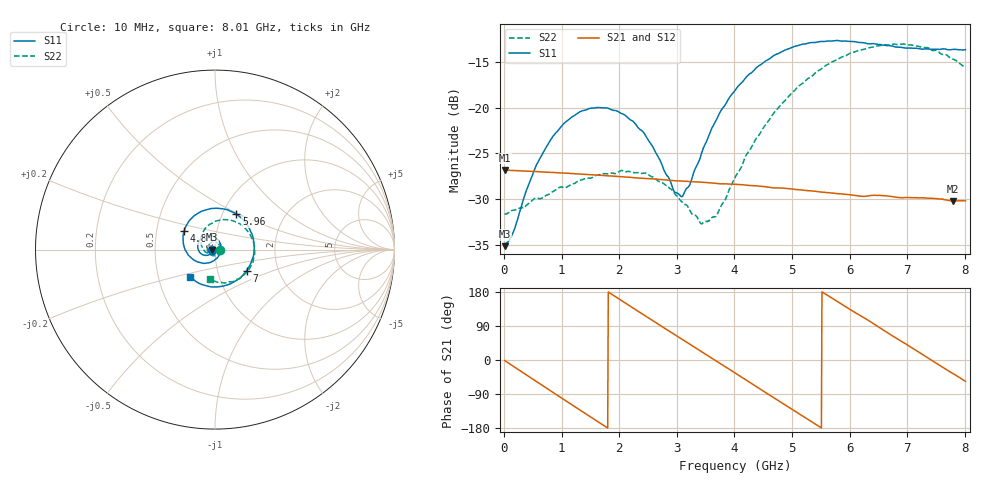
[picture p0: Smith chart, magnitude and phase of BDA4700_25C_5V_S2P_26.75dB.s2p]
!Agilent Technologies,E5071B,MY42404982,A.09.10
!Date: Mon Oct 20 13:39:58 2025
!Data & Calibration Information:
!Freq	S11:SOLT2(ON)	S21:SOLT2(ON)	S12:SOLT2(ON)	S22:SOLT2(ON)
# Hz S RI R 50
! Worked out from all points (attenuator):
!   801 points, 10 MHz to 8.01 GHz, reference 50 ohm
!   highest |S21| = -26.82 dB at 10 MHz (marker M1); lowest = -30.2 dB at 7.8 GHz (marker M2)
!   lowest |S11| = -35.2 dB at 10 MHz (marker M3), VSWR 1.04, Z = 48.3 - j0.102 ohm
!   |S11| at or under -10 dB: start of sweep to end of sweep
!   |S22| runs from -32.7 to -13.0 dB; largest |S21 - S12| = 0.00038
!   S11 on the Smith chart (normalised r, x): 10 MHz: 0.97, -0.00; 4.8 GHz: 0.69, +0.15; 5.96 GHz: 1.16, +0.48; 7 GHz: 1.38, -0.34; 8.01 GHz: 0.73, -0.23
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1e7  -0.0174 -0.00105  0.0456 -0.000973  0.0456 -0.00104  0.0261 -0.000789
1.5e8  -0.0184 -0.00909  0.0436 -0.0121  0.0436 -0.0121  0.0264 -0.00716
4.3e8  -0.0284 -0.0253  0.0324 -0.031  0.0325 -0.0309  0.0196 -0.0226
7.1e8  -0.0491 -0.0326  0.0141 -0.0421  0.014 -0.0421  0.00522 -0.0324
1.35e9  -0.0956 0.0061  -0.0306 -0.0305  -0.0306 -0.0305  -0.036 -0.0178
2.08e9  -0.051 0.0761  -0.0372 0.019  -0.0372 0.019  -0.0297 0.0335
2.42e9  -0.00594 0.073  -0.0203 0.0357  -0.0203 0.0357  -0.00495 0.0434
2.68e9  0.0215 0.049  -0.0031 0.0404  -0.0031 0.0404  0.0128 0.0374
2.95e9  0.0331 0.0112  0.0148 0.037  0.0148 0.0369  0.0251 0.0233
3.1e9  0.0304 -0.0119  0.0234 0.0319  0.0234 0.032  0.028 0.0115
3.41e9  0.00297 -0.0534  0.0358 0.0158  0.0358 0.0158  0.0203 -0.0115
3.54e9  -0.0157 -0.0662  0.0381 0.00757  0.0381 0.00752  0.0129 -0.0202
3.7e9  -0.045 -0.0748  0.0383 -0.00278  0.0383 -0.0029  -0.000747 -0.0259
4.01e9  -0.1061 -0.0642  0.0315 -0.0213  0.0315 -0.0213  -0.0323 -0.0257
4.8e9  -0.1722 0.1018  -0.0128 -0.034  -0.0127 -0.034  -0.078 0.0672
5.35e9  -0.0688 0.2157  -0.0336 -0.00972  -0.0336 -0.0098  -0.0152 0.1479
5.96e9  0.1191 0.1971  -0.0248 0.0224  -0.0249 0.0223  0.1217 0.1512
6.68e9  0.2175 -0.0148  0.0113 0.0307  0.0113 0.0307  0.2197 -0.000102
7e9  0.1758 -0.1172  0.0246 0.0207  0.0247 0.0206  0.2029 -0.0857
7.41e9  0.0597 -0.1994  0.0319 0.000359  0.0319 0.000285  0.1259 -0.1647
7.8e9  -0.0769 -0.1933  0.0248 -0.0182  0.0248 -0.0184  0.0202 -0.1823
8.01e9  -0.1378 -0.1548  0.0171 -0.0257  0.0173 -0.0257  -0.0305 -0.1618
